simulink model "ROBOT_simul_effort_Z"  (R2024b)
settings: Solver=VariableStepAuto  StartTime=0.0  StopTime=5  RelTol=1e-3
undefined symbols (not defined in the file): a, ARRIERE_Defaut_sldprt, avant01_Defaut_sldprt, avant02_Defaut_sldprt, avant03_Defaut_sldprt, avant1_Defaut_sldprt, AXE, BASE_Defaut_sldprt, BIELLE, BIELLE_Defaut_sldprt, BRAS_Defaut_sldprt, bras_Defaut_sldprt, C_Realiste_sldprt, CABLE_Defaut_sldprt, cable_Defaut_sldprt, CACHE_Defaut_sldprt, CARTE, carte_Defaut_sldprt, CARTER, carter, CHC, CODEUR_Defaut_sldprt, cruciforme, cylindrique, deg, Drive, Fichiers, Fichiers_Matlab_sujetA, FIXATION, fixation_Defaut_sldprt, H, HEXAGONALE_Defaut_sldprt, joint_Defaut_sldprt, kg, m, M4, M4_Defaut_sldprt, manette1_Defaut_sldprt, manette2_Defaut_sldprt, MATLAB, Matlab, matlab_Defaut_sldprt, mm, modif, MOTEUR_Defaut_sldprt, N, NEZ_Defaut_sldprt, nom, palier, PARALLELOGRAMME_Defaut_sldprt, petite, plaque, rad, Ressort, Rondelle, ROTOR_Defaut_sldprt, s, SET, simple, socle_Defaut_sldprt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
libraries: sm_lib x463, fl_lib x45, nesl_utility x27, simulink x2
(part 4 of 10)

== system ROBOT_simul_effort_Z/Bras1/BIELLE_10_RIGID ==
  AXE_BIELLE_1_RIGID : Subsystem
  AXE_BIELLE_2_RIGID : Subsystem
  BIELLE_PARALLELOGRAMME_1_RIGID : Subsystem
  ReferenceFrame : sm_lib/Frames and Transforms/Reference Frame
  Transform : sm_lib/Frames and Transforms/Rigid Transform  RotationMethod=ArbitraryAxis  FollAlignAxisA=+X  BaseAlignAxisA=+Y  FollAlignAxisB=+Y  BaseAlignAxisB=+Z  RotationStandardAxis=+Z  RotationAngle=2.0943951023931957  RotationAngleUnits=rad  RotationArbitraryAxis=[0.57735026918962573 -0.57735026918962573 0.57735026918962562]  RotationSequenceAxes=FollowerAxes  RotationSequence=XYX  RotationSequenceAngles=[0 0 0]  RotationSequenceAnglesUnits=deg  RotationMatrix=[1 0 0; 0 1 0; 0 0 1]  Quaternion=[1 0 0 0]  TranslationMethod=Cartesian  TranslationCartesianOffset=[-181.1287710013672 12.999999999999993 -105.75000000000001]  TranslationCartesianOffsetUnits=mm  TranslationStandardAxis=+Z  TranslationStandardOffset=0  TranslationStandardOffsetUnits=mm  TranslationROffset=0  TranslationROffsetUnits=m  TranslationThetaOffset=0  TranslationThetaOffsetUnits=deg  TranslationZOffset=0  TranslationZOffsetUnits=m
  Transform1 : sm_lib/Frames and Transforms/Rigid Transform  RotationMethod=ArbitraryAxis  FollAlignAxisA=+X  BaseAlignAxisA=+Y  FollAlignAxisB=+Y  BaseAlignAxisB=+Z  RotationStandardAxis=+Z  RotationAngle=2.0943951023931953  RotationAngleUnits=rad  RotationArbitraryAxis=[0.57735026918962584 -0.57735026918962584 0.57735026918962584]  RotationSequenceAxes=FollowerAxes  RotationSequence=XYX  RotationSequenceAngles=[0 0 0]  RotationSequenceAnglesUnits=deg  RotationMatrix=[1 0 0; 0 1 0; 0 0 1]  Quaternion=[1 0 0 0]  TranslationMethod=Cartesian  TranslationCartesianOffset=[-181.12877100136717 13.000000000000004 -3.249999999999996]  TranslationCartesianOffsetUnits=mm  TranslationStandardAxis=+Z  TranslationStandardOffset=0  TranslationStandardOffsetUnits=mm  TranslationROffset=0  TranslationROffsetUnits=m  TranslationThetaOffset=0  TranslationThetaOffsetUnits=deg  TranslationZOffset=0  TranslationZOffsetUnits=m
  Transform2 : sm_lib/Frames and Transforms/Rigid Transform  RotationMethod=ArbitraryAxis  FollAlignAxisA=+X  BaseAlignAxisA=+Y  FollAlignAxisB=+Y  BaseAlignAxisB=+Z  RotationStandardAxis=+Z  RotationAngle=3.1415926535897931  RotationAngleUnits=rad  RotationArbitraryAxis=[-0.70710678118654746 0.70710678118654768 0]  RotationSequenceAxes=FollowerAxes  RotationSequence=XYX  RotationSequenceAngles=[0 0 0]  RotationSequenceAnglesUnits=deg  RotationMatrix=[1 0 0; 0 1 0; 0 0 1]  Quaternion=[1 0 0 0]  TranslationMethod=Cartesian  TranslationCartesianOffset=[-178.12877100136717 5.0000000000000115 -54.500000000000007]  TranslationCartesianOffsetUnits=mm  TranslationStandardAxis=+Z  TranslationStandardOffset=0  TranslationStandardOffsetUnits=mm  TranslationROffset=0  TranslationROffsetUnits=m  TranslationThetaOffset=0  TranslationThetaOffsetUnits=deg  TranslationZOffset=0  TranslationZOffsetUnits=m
  Transform3 : sm_lib/Frames and Transforms/Rigid Transform  RotationMethod=ArbitraryAxis  FollAlignAxisA=+X  BaseAlignAxisA=+Y  FollAlignAxisB=+Y  BaseAlignAxisB=+Z  RotationStandardAxis=+Z  RotationAngle=1.7602050674842988  RotationAngleUnits=rad  RotationArbitraryAxis=[-0.82650316451596495 -0.3980530863120495 -0.3980530863120495]  RotationSequenceAxes=FollowerAxes  RotationSequence=XYX  RotationSequenceAngles=[0 0 0]  RotationSequenceAnglesUnits=deg  RotationMatrix=[1 0 0; 0 1 0; 0 0 1]  Quaternion=[1 0 0 0]  TranslationMethod=Cartesian  TranslationCartesianOffset=[-181.1287710013672 4.999999999999984 -105.75000000000001]  TranslationCartesianOffsetUnits=mm  TranslationStandardAxis=+Z  TranslationStandardOffset=0  TranslationStandardOffsetUnits=mm  TranslationROffset=0  TranslationROffsetUnits=m  TranslationThetaOffset=0  TranslationThetaOffsetUnits=deg  TranslationZOffset=0  TranslationZOffsetUnits=m
  Transform4 : sm_lib/Frames and Transforms/Rigid Transform  RotationMethod=ArbitraryAxis  FollAlignAxisA=+X  BaseAlignAxisA=+Y  FollAlignAxisB=+Y  BaseAlignAxisB=+Z  RotationStandardAxis=+Z  RotationAngle=1.7602050674842997  RotationAngleUnits=rad  RotationArbitraryAxis=[-0.82650316451596506 -0.39805308631204933 -0.39805308631204933]  RotationSequenceAxes=FollowerAxes  RotationSequence=XYX  RotationSequenceAngles=[0 0 0]  RotationSequenceAnglesUnits=deg  RotationMatrix=[1 0 0; 0 1 0; 0 0 1]  Quaternion=[1 0 0 0]  TranslationMethod=Cartesian  TranslationCartesianOffset=[-181.12877100136717 5.0000000000000115 -3.249999999999996]  TranslationCartesianOffsetUnits=mm  TranslationStandardAxis=+Z  TranslationStandardOffset=0  TranslationStandardOffsetUnits=mm  TranslationROffset=0  TranslationROffsetUnits=m  TranslationThetaOffset=0  TranslationThetaOffsetUnits=deg  TranslationZOffset=0  TranslationZOffsetUnits=m
  F1 : PMIOPort  Side=Right
  F : PMIOPort  Port=2  Side=Left
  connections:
  Transform/LConn1 -- ReferenceFrame/RConn1 -- Transform3/LConn1 -- Transform4/LConn1 -- Transform2/LConn1 -- Transform1/LConn1
  Transform/RConn1 -- F/RConn1
  Transform1/RConn1 -- F1/RConn1
  BIELLE_PARALLELOGRAMME_1_RIGID/LConn1 -- Transform2/RConn1
  AXE_BIELLE_1_RIGID/LConn1 -- Transform3/RConn1
  AXE_BIELLE_2_RIGID/LConn1 -- Transform4/RConn1

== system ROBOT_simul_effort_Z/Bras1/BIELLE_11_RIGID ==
  AXE_BIELLE_1_RIGID : Subsystem
  AXE_BIELLE_2_RIGID : Subsystem
  BIELLE_PARALLELOGRAMME_1_RIGID : Subsystem
  ReferenceFrame : sm_lib/Frames and Transforms/Reference Frame
  Transform : sm_lib/Frames and Transforms/Rigid Transform  RotationMethod=ArbitraryAxis  FollAlignAxisA=+X  BaseAlignAxisA=+Y  FollAlignAxisB=+Y  BaseAlignAxisB=+Z  RotationStandardAxis=+Z  RotationAngle=2.0943951023931962  RotationAngleUnits=rad  RotationArbitraryAxis=[0.57735026918962595 -0.57735026918962562 0.57735026918962562]  RotationSequenceAxes=FollowerAxes  RotationSequence=XYX  RotationSequenceAngles=[0 0 0]  RotationSequenceAnglesUnits=deg  RotationMatrix=[1 0 0; 0 1 0; 0 0 1]  Quaternion=[1 0 0 0]  TranslationMethod=Cartesian  TranslationCartesianOffset=[-181.12877100136717 13.000000000000018 -105.75000000000001]  TranslationCartesianOffsetUnits=mm  TranslationStandardAxis=+Z  TranslationStandardOffset=0  TranslationStandardOffsetUnits=mm  TranslationROffset=0  TranslationROffsetUnits=m  TranslationThetaOffset=0  TranslationThetaOffsetUnits=deg  TranslationZOffset=0  TranslationZOffsetUnits=m
  Transform1 : sm_lib/Frames and Transforms/Rigid Transform  RotationMethod=ArbitraryAxis  FollAlignAxisA=+X  BaseAlignAxisA=+Y  FollAlignAxisB=+Y  BaseAlignAxisB=+Z  RotationStandardAxis=+Z  RotationAngle=2.0943951023931957  RotationAngleUnits=rad  RotationArbitraryAxis=[0.57735026918962573 -0.57735026918962562 0.57735026918962595]  RotationSequenceAxes=FollowerAxes  RotationSequence=XYX  RotationSequenceAngles=[0 0 0]  RotationSequenceAnglesUnits=deg  RotationMatrix=[1 0 0; 0 1 0; 0 0 1]  Quaternion=[1 0 0 0]  TranslationMethod=Cartesian  TranslationCartesianOffset=[-181.12877100136714 13.000000000000014 -3.2499999999999889]  TranslationCartesianOffsetUnits=mm  TranslationStandardAxis=+Z  TranslationStandardOffset=0  TranslationStandardOffsetUnits=mm  TranslationROffset=0  TranslationROffsetUnits=m  TranslationThetaOffset=0  TranslationThetaOffsetUnits=deg  TranslationZOffset=0  TranslationZOffsetUnits=m
  Transform2 : sm_lib/Frames and Transforms/Rigid Transform  RotationMethod=ArbitraryAxis  FollAlignAxisA=+X  BaseAlignAxisA=+Y  FollAlignAxisB=+Y  BaseAlignAxisB=+Z  RotationStandardAxis=+Z  RotationAngle=3.1415926535897931  RotationAngleUnits=rad  RotationArbitraryAxis=[-0.70710678118654746 0.70710678118654757 0]  RotationSequenceAxes=FollowerAxes  RotationSequence=XYX  RotationSequenceAngles=[0 0 0]  RotationSequenceAnglesUnits=deg  RotationMatrix=[1 0 0; 0 1 0; 0 0 1]  Quaternion=[1 0 0 0]  TranslationMethod=Cartesian  TranslationCartesianOffset=[-178.12877100136714 5.0000000000000044 -54.500000000000007]  TranslationCartesianOffsetUnits=mm  TranslationStandardAxis=+Z  TranslationStandardOffset=0  TranslationStandardOffsetUnits=mm  TranslationROffset=0  TranslationROffsetUnits=m  TranslationThetaOffset=0  TranslationThetaOffsetUnits=deg  TranslationZOffset=0  TranslationZOffsetUnits=m
  Transform3 : sm_lib/Frames and Transforms/Rigid Transform  RotationMethod=ArbitraryAxis  FollAlignAxisA=+X  BaseAlignAxisA=+Y  FollAlignAxisB=+Y  BaseAlignAxisB=+Z  RotationStandardAxis=+Z  RotationAngle=1.7602050674842991  RotationAngleUnits=rad  RotationArbitraryAxis=[-0.82650316451596495 -0.3980530863120495 -0.39805308631204944]  RotationSequenceAxes=FollowerAxes  RotationSequence=XYX  RotationSequenceAngles=[0 0 0]  RotationSequenceAnglesUnits=deg  RotationMatrix=[1 0 0; 0 1 0; 0 0 1]  Quaternion=[1 0 0 0]  TranslationMethod=Cartesian  TranslationCartesianOffset=[-181.12877100136717 5.0000000000000044 -105.75000000000001]  TranslationCartesianOffsetUnits=mm  TranslationStandardAxis=+Z  TranslationStandardOffset=0  TranslationStandardOffsetUnits=mm  TranslationROffset=0  TranslationROffsetUnits=m  TranslationThetaOffset=0  TranslationThetaOffsetUnits=deg  TranslationZOffset=0  TranslationZOffsetUnits=m
  Transform4 : sm_lib/Frames and Transforms/Rigid Transform  RotationMethod=ArbitraryAxis  FollAlignAxisA=+X  BaseAlignAxisA=+Y  FollAlignAxisB=+Y  BaseAlignAxisB=+Z  RotationStandardAxis=+Z  RotationAngle=1.7602050674842995  RotationAngleUnits=rad  RotationArbitraryAxis=[-0.82650316451596506 -0.39805308631204939 -0.39805308631204933]  RotationSequenceAxes=FollowerAxes  RotationSequence=XYX  RotationSequenceAngles=[0 0 0]  RotationSequenceAnglesUnits=deg  RotationMatrix=[1 0 0; 0 1 0; 0 0 1]  Quaternion=[1 0 0 0]  TranslationMethod=Cartesian  TranslationCartesianOffset=[-181.12877100136714 5.0000000000000044 -3.2499999999999889]  TranslationCartesianOffsetUnits=mm  TranslationStandardAxis=+Z  TranslationStandardOffset=0  TranslationStandardOffsetUnits=mm  TranslationROffset=0  TranslationROffsetUnits=m  TranslationThetaOffset=0  TranslationThetaOffsetUnits=deg  TranslationZOffset=0  TranslationZOffsetUnits=m
  F1 : PMIOPort  Side=Right
  F : PMIOPort  Port=2  Side=Left
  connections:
  Transform/LConn1 -- ReferenceFrame/RConn1 -- Transform3/LConn1 -- Transform4/LConn1 -- Transform2/LConn1 -- Transform1/LConn1
  Transform/RConn1 -- F/RConn1
  Transform1/RConn1 -- F1/RConn1
  BIELLE_PARALLELOGRAMME_1_RIGID/LConn1 -- Transform2/RConn1
  AXE_BIELLE_1_RIGID/LConn1 -- Transform3/RConn1
  AXE_BIELLE_2_RIGID/LConn1 -- Transform4/RConn1

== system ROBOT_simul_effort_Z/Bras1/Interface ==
  Angular Velocity Source : fl_lib/Mechanical/Mechanical Sources/Ideal Angular Velocity Source
  Torque Sensor : fl_lib/Mechanical/Mechanical Sensors/Ideal Torque Sensor
  C : PMIOPort  Side=Left
  T : PMIOPort  Port=2  Side=Right
  w : PMIOPort  Port=3  Side=Right
  R : PMIOPort  Port=4  Side=Left
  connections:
  R/RConn1 -- Angular Velocity Source/LConn1
  Torque Sensor/LConn1 -- Angular Velocity Source/RConn2
  Torque Sensor/RConn2 -- T/RConn1
  C/RConn1 -- Torque Sensor/RConn1
  Angular Velocity Source/RConn1 -- w/RConn1

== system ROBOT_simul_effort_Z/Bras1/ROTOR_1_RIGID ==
  CODEUR_1_RIGID : Subsystem
  ROTOR_1_RIGID : Subsystem
  ReferenceFrame : sm_lib/Frames and Transforms/Reference Frame
  Transform : sm_lib/Frames and Transforms/Rigid Transform  RotationMethod=ArbitraryAxis  FollAlignAxisA=+X  BaseAlignAxisA=+Y  FollAlignAxisB=+Y  BaseAlignAxisB=+Z  RotationStandardAxis=+Z  RotationAngle=2.0943951023931953  RotationAngleUnits=rad  RotationArbitraryAxis=[0.57735026918962595 0.57735026918962562 0.57735026918962562]  RotationSequenceAxes=FollowerAxes  RotationSequence=XYX  RotationSequenceAngles=[0 0 0]  RotationSequenceAnglesUnits=deg  RotationMatrix=[1 0 0; 0 1 0; 0 0 1]  Quaternion=[1 0 0 0]  TranslationMethod=Cartesian  TranslationCartesianOffset=[29.900000000000013 -3.5527136788005009e-15 2.2204460492503131e-14]  TranslationCartesianOffsetUnits=mm  TranslationStandardAxis=+Z  TranslationStandardOffset=0  TranslationStandardOffsetUnits=mm  TranslationROffset=0  TranslationROffsetUnits=m  TranslationThetaOffset=0  TranslationThetaOffsetUnits=deg  TranslationZOffset=0  TranslationZOffsetUnits=m
  Transform1 : sm_lib/Frames and Transforms/Rigid Transform  RotationMethod=ArbitraryAxis  FollAlignAxisA=+X  BaseAlignAxisA=+Y  FollAlignAxisB=+Y  BaseAlignAxisB=+Z  RotationStandardAxis=+Z  RotationAngle=1.9381695666920586  RotationAngleUnits=rad  RotationArbitraryAxis=[0.51405666735189148 -0.51405666735189148 0.68665237602598705]  RotationSequenceAxes=FollowerAxes  RotationSequence=XYX  RotationSequenceAngles=[0 0 0]  RotationSequenceAnglesUnits=deg  RotationMatrix=[1 0 0; 0 1 0; 0 0 1]  Quaternion=[1 0 0 0]  TranslationMethod=Cartesian  TranslationCartesianOffset=[30.899999999999981 0 0]  TranslationCartesianOffsetUnits=mm  TranslationStandardAxis=+Z  TranslationStandardOffset=0  TranslationStandardOffsetUnits=mm  TranslationROffset=0  TranslationROffsetUnits=m  TranslationThetaOffset=0  TranslationThetaOffsetUnits=deg  TranslationZOffset=0  TranslationZOffsetUnits=m
  Transform2 : sm_lib/Frames and Transforms/Rigid Transform  RotationMethod=ArbitraryAxis  FollAlignAxisA=+X  BaseAlignAxisA=+Y  FollAlignAxisB=+Y  BaseAlignAxisB=+Z  RotationStandardAxis=+Z  RotationAngle=1.624664356272121  RotationAngleUnits=rad  RotationArbitraryAxis=[-0.22603347840136145 0.22603347840136123 0.94753244444903439]  RotationSequenceAxes=FollowerAxes  RotationSequence=XYX  RotationSequenceAngles=[0 0 0]  RotationSequenceAnglesUnits=deg  RotationMatrix=[1 0 0; 0 1 0; 0 0 1]  Quaternion=[1 0 0 0]  TranslationMethod=Cartesian  TranslationCartesianOffset=[-36.399999999999999 0 0]  TranslationCartesianOffsetUnits=mm  TranslationStandardAxis=+Z  TranslationStandardOffset=0  TranslationStandardOffsetUnits=mm  TranslationROffset=0  TranslationROffsetUnits=m  TranslationThetaOffset=0  TranslationThetaOffsetUnits=deg  TranslationZOffset=0  TranslationZOffsetUnits=m
  F : PMIOPort  Side=Left
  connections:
  Transform/LConn1 -- ReferenceFrame/RConn1 -- Transform1/LConn1 -- Transform2/LConn1
  Transform/RConn1 -- F/RConn1
  ROTOR_1_RIGID/LConn1 -- Transform1/RConn1
  CODEUR_1_RIGID/LConn1 -- Transform2/RConn1

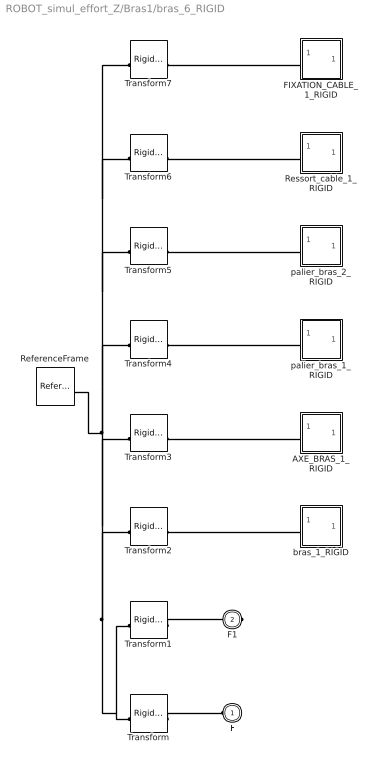
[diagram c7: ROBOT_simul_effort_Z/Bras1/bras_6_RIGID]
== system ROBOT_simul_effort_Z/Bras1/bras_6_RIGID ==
  AXE_BRAS_1_RIGID : Subsystem
  FIXATION_CABLE_1_RIGID : Subsystem
  ReferenceFrame : sm_lib/Frames and Transforms/Reference Frame
  Ressort_cable_1_RIGID : Subsystem
  Transform : sm_lib/Frames and Transforms/Rigid Transform  RotationMethod=ArbitraryAxis  FollAlignAxisA=+X  BaseAlignAxisA=+Y  FollAlignAxisB=+Y  BaseAlignAxisB=+Z  RotationStandardAxis=+Z  RotationAngle=2.0943951023931957  RotationAngleUnits=rad  RotationArbitraryAxis=[-0.57735026918962551 -0.57735026918962595 0.57735026918962573]  RotationSequenceAxes=FollowerAxes  RotationSequence=XYX  RotationSequenceAngles=[0 0 0]  RotationSequenceAnglesUnits=deg  RotationMatrix=[1 0 0; 0 1 0; 0 0 1]  Quaternion=[1 0 0 0]  TranslationMethod=Cartesian  TranslationCartesianOffset=[-97.415569487383038 39.82561820207529 -20.980989744699272]  TranslationCartesianOffsetUnits=mm  TranslationStandardAxis=+Z  TranslationStandardOffset=0  TranslationStandardOffsetUnits=mm  TranslationROffset=0  TranslationROffsetUnits=m  TranslationThetaOffset=0  TranslationThetaOffsetUnits=deg  TranslationZOffset=0  TranslationZOffsetUnits=m
  Transform1 : sm_lib/Frames and Transforms/Rigid Transform  RotationMethod=ArbitraryAxis  FollAlignAxisA=+X  BaseAlignAxisA=+Y  FollAlignAxisB=+Y  BaseAlignAxisB=+Z  RotationStandardAxis=+Z  RotationAngle=2.0943951023931953  RotationAngleUnits=rad  RotationArbitraryAxis=[0.57735026918962584 0.57735026918962584 0.57735026918962584]  RotationSequenceAxes=FollowerAxes  RotationSequence=XYX  RotationSequenceAngles=[0 0 0]  RotationSequenceAnglesUnits=deg  RotationMatrix=[1 0 0; 0 1 0; 0 0 1]  Quaternion=[1 0 0 0]  TranslationMethod=Cartesian  TranslationCartesianOffset=[-176.59192436800635 99.825618202078147 -20.980989744703663]  TranslationCartesianOffsetUnits=mm  TranslationStandardAxis=+Z  TranslationStandardOffset=0  TranslationStandardOffsetUnits=mm  TranslationROffset=0  TranslationROffsetUnits=m  TranslationThetaOffset=0  TranslationThetaOffsetUnits=deg  TranslationZOffset=0  TranslationZOffsetUnits=m
  Transform2 : sm_lib/Frames and Transforms/Rigid Transform  RotationMethod=ArbitraryAxis  FollAlignAxisA=+X  BaseAlignAxisA=+Y  FollAlignAxisB=+Y  BaseAlignAxisB=+Z  RotationStandardAxis=+Z  RotationAngle=1.5707963267948968  RotationAngleUnits=rad  RotationArbitraryAxis=[-0 -1 -0]  RotationSequenceAxes=FollowerAxes  RotationSequence=XYX  RotationSequenceAngles=[0 0 0]  RotationSequenceAnglesUnits=deg  RotationMatrix=[1 0 0; 0 1 0; 0 0 1]  Quaternion=[1 0 0 0]  TranslationMethod=Cartesian  TranslationCartesianOffset=[-166.59192436800635 39.825618202078147 -20.98098974470366]  TranslationCartesianOffsetUnits=mm  TranslationStandardAxis=+Z  TranslationStandardOffset=0  TranslationStandardOffsetUnits=mm  TranslationROffset=0  TranslationROffsetUnits=m  TranslationThetaOffset=0  TranslationThetaOffsetUnits=deg  TranslationZOffset=0  TranslationZOffsetUnits=m
  Transform3 : sm_lib/Frames and Transforms/Rigid Transform  RotationMethod=ArbitraryAxis  FollAlignAxisA=+X  BaseAlignAxisA=+Y  FollAlignAxisB=+Y  BaseAlignAxisB=+Z  RotationStandardAxis=+Z  RotationAngle=1.5707963267948968  RotationAngleUnits=rad  RotationArbitraryAxis=[0 1 0]  RotationSequenceAxes=FollowerAxes  RotationSequence=XYX  RotationSequenceAngles=[0 0 0]  RotationSequenceAnglesUnits=deg  RotationMatrix=[1 0 0; 0 1 0; 0 0 1]  Quaternion=[1 0 0 0]  TranslationMethod=Cartesian  TranslationCartesianOffset=[-166.59192436800635 39.825618202078147 -20.98098974470366]  TranslationCartesianOffsetUnits=mm  TranslationStandardAxis=+Z  TranslationStandardOffset=0  TranslationStandardOffsetUnits=mm  TranslationROffset=0  TranslationROffsetUnits=m  TranslationThetaOffset=0  TranslationThetaOffsetUnits=deg  TranslationZOffset=0  TranslationZOffsetUnits=m
  Transform4 : sm_lib/Frames and Transforms/Rigid Transform  RotationMethod=None  FollAlignAxisA=+X  BaseAlignAxisA=+Y  FollAlignAxisB=+Y  BaseAlignAxisB=+Z  RotationStandardAxis=+Z  RotationAngle=0  RotationAngleUnits=deg  RotationArbitraryAxis=[0 0 1]  RotationSequenceAxes=FollowerAxes  RotationSequence=XYX  RotationSequenceAngles=[0 0 0]  RotationSequenceAnglesUnits=deg  RotationMatrix=[1 0 0; 0 1 0; 0 0 1]  Quaternion=[1 0 0 0]  TranslationMethod=None  TranslationCartesianOffset=[0 0 0]  TranslationCartesianOffsetUnits=m  TranslationStandardAxis=+Z  TranslationStandardOffset=0  TranslationStandardOffsetUnits=m  TranslationROffset=0  TranslationROffsetUnits=m  TranslationThetaOffset=0  TranslationThetaOffsetUnits=deg  TranslationZOffset=0  TranslationZOffsetUnits=m
  Transform5 : sm_lib/Frames and Transforms/Rigid Transform  RotationMethod=ArbitraryAxis  FollAlignAxisA=+X  BaseAlignAxisA=+Y  FollAlignAxisB=+Y  BaseAlignAxisB=+Z  RotationStandardAxis=+Z  RotationAngle=3.1415926535897931  RotationAngleUnits=rad  RotationArbitraryAxis=[0 0.83121877946981937 -0.55594544755461728]  RotationSequenceAxes=FollowerAxes  RotationSequence=XYX  RotationSequenceAngles=[0 0 0]  RotationSequenceAnglesUnits=deg  RotationMatrix=[1 0 0; 0 1 0; 0 0 1]  Quaternion=[1 0 0 0]  TranslationMethod=Cartesian  TranslationCartesianOffset=[-333.18384873601275 5.2270863233389582 7.8152493791980238]  TranslationCartesianOffsetUnits=mm  TranslationStandardAxis=+Z  TranslationStandardOffset=0  TranslationStandardOffsetUnits=mm  TranslationROffset=0  TranslationROffsetUnits=m  TranslationThetaOffset=0  TranslationThetaOffsetUnits=deg  TranslationZOffset=0  TranslationZOffsetUnits=m
  Transform6 : sm_lib/Frames and Transforms/Rigid Transform  RotationMethod=ArbitraryAxis  FollAlignAxisA=+X  BaseAlignAxisA=+Y  FollAlignAxisB=+Y  BaseAlignAxisB=+Z  RotationStandardAxis=+Z  RotationAngle=1.5707963267948968  RotationAngleUnits=rad  RotationArbitraryAxis=[1 0 0]  RotationSequenceAxes=FollowerAxes  RotationSequence=XYX  RotationSequenceAngles=[0 0 0]  RotationSequenceAnglesUnits=deg  RotationMatrix=[1 0 0; 0 1 0; 0 0 1]  Quaternion=[1 0 0 0]  TranslationMethod=Cartesian  TranslationCartesianOffset=[-166.59192436800637 17.182941135267072 -24.980989744703663]  TranslationCartesianOffsetUnits=mm  TranslationStandardAxis=+Z  TranslationStandardOffset=0  TranslationStandardOffsetUnits=mm  TranslationROffset=0  TranslationROffsetUnits=m  TranslationThetaOffset=0  TranslationThetaOffsetUnits=deg  TranslationZOffset=0  TranslationZOffsetUnits=m
  Transform7 : sm_lib/Frames and Transforms/Rigid Transform  RotationMethod=ArbitraryAxis  FollAlignAxisA=+X  BaseAlignAxisA=+Y  FollAlignAxisB=+Y  BaseAlignAxisB=+Z  RotationStandardAxis=+Z  RotationAngle=1.0159852938148253  RotationAngleUnits=rad  RotationArbitraryAxis=[-1 0 0]  RotationSequenceAxes=FollowerAxes  RotationSequence=XYX  RotationSequenceAngles=[0 0 0]  RotationSequenceAnglesUnits=deg  RotationMatrix=[1 0 0; 0 1 0; 0 0 1]  Quaternion=[1 0 0 0]  TranslationMethod=Cartesian  TranslationCartesianOffset=[-172.59192436800637 90.586314327933906 3.4188407632840327]  TranslationCartesianOffsetUnits=mm  TranslationStandardAxis=+Z  TranslationStandardOffset=0  TranslationStandardOffsetUnits=mm  TranslationROffset=0  TranslationROffsetUnits=m  TranslationThetaOffset=0  TranslationThetaOffsetUnits=deg  TranslationZOffset=0  TranslationZOffsetUnits=m
  bras_1_RIGID : Subsystem
  palier_bras_1_RIGID : Subsystem
  palier_bras_2_RIGID : Subsystem
  F : PMIOPort  Side=Left
  F1 : PMIOPort  Port=2  Side=Right
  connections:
  Transform/LConn1 -- ReferenceFrame/RConn1 -- Transform6/LConn1 -- Transform7/LConn1 -- Transform5/LConn1 -- Transform4/LConn1 -- Transform3/LConn1 -- Transform2/LConn1 -- Transform1/LConn1
  Transform/RConn1 -- F/RConn1
  Transform1/RConn1 -- F1/RConn1
  Transform2/RConn1 -- bras_1_RIGID/LConn1
  AXE_BRAS_1_RIGID/LConn1 -- Transform3/RConn1
  Transform4/RConn1 -- palier_bras_1_RIGID/LConn1
  Transform5/RConn1 -- palier_bras_2_RIGID/LConn1
  Ressort_cable_1_RIGID/LConn1 -- Transform6/RConn1
  FIXATION_CABLE_1_RIGID/LConn1 -- Transform7/RConn1

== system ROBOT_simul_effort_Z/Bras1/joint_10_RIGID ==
  AXE_BRAS_1_RIGID : Subsystem
  ReferenceFrame : sm_lib/Frames and Transforms/Reference Frame
  Transform : sm_lib/Frames and Transforms/Rigid Transform  RotationMethod=ArbitraryAxis  FollAlignAxisA=+X  BaseAlignAxisA=+Y  FollAlignAxisB=+Y  BaseAlignAxisB=+Z  RotationStandardAxis=+Z  RotationAngle=1.9754511492118261  RotationAngleUnits=rad  RotationArbitraryAxis=[-0.53149434051907762 -0.53149434051907807 -0.65956616953295977]  RotationSequenceAxes=FollowerAxes  RotationSequence=XYX  RotationSequenceAngles=[0 0 0]  RotationSequenceAnglesUnits=deg  RotationMatrix=[1 0 0; 0 1 0; 0 0 1]  Quaternion=[1 0 0 0]  TranslationMethod=Cartesian  TranslationCartesianOffset=[-153.62772197331242 116.19029839316632 -133.8263224253264]  TranslationCartesianOffsetUnits=mm  TranslationStandardAxis=+Z  TranslationStandardOffset=0  TranslationStandardOffsetUnits=mm  TranslationROffset=0  TranslationROffsetUnits=m  TranslationThetaOffset=0  TranslationThetaOffsetUnits=deg  TranslationZOffset=0  TranslationZOffsetUnits=m
  Transform1 : sm_lib/Frames and Transforms/Rigid Transform  RotationMethod=ArbitraryAxis  FollAlignAxisA=+X  BaseAlignAxisA=+Y  FollAlignAxisB=+Y  BaseAlignAxisB=+Z  RotationStandardAxis=+Z  RotationAngle=2.2221940470110657  RotationAngleUnits=rad  RotationArbitraryAxis=[0.61437017396793003 -0.61437017396792981 0.49507431631749077]  RotationSequenceAxes=FollowerAxes  RotationSequence=XYX  RotationSequenceAngles=[0 0 0]  RotationSequenceAnglesUnits=deg  RotationMatrix=[1 0 0; 0 1 0; 0 0 1]  Quaternion=[1 0 0 0]  TranslationMethod=Cartesian  TranslationCartesianOffset=[-181.62772197331248 131.82453775326121 -130.42476989284125]  TranslationCartesianOffsetUnits=mm  TranslationStandardAxis=+Z  TranslationStandardOffset=0  TranslationStandardOffsetUnits=mm  TranslationROffset=0  TranslationROffsetUnits=m  TranslationThetaOffset=0  TranslationThetaOffsetUnits=deg  TranslationZOffset=0  TranslationZOffsetUnits=m
  Transform2 : sm_lib/Frames and Transforms/Rigid Transform  RotationMethod=ArbitraryAxis  FollAlignAxisA=+X  BaseAlignAxisA=+Y  FollAlignAxisB=+Y  BaseAlignAxisB=+Z  RotationStandardAxis=+Z  RotationAngle=2.0943951023931957  RotationAngleUnits=rad  RotationArbitraryAxis=[0.57735026918962551 0.57735026918962584 0.57735026918962595]  RotationSequenceAxes=FollowerAxes  RotationSequence=XYX  RotationSequenceAngles=[0 0 0]  RotationSequenceAnglesUnits=deg  RotationMatrix=[1 0 0; 0 1 0; 0 0 1]  Quaternion=[1 0 0 0]  TranslationMethod=Cartesian  TranslationCartesianOffset=[-177.62772197331233 126.39913469761095 -143.1183707091472]  TranslationCartesianOffsetUnits=mm  TranslationStandardAxis=+Z  TranslationStandardOffset=0  TranslationStandardOffsetUnits=mm  TranslationROffset=0  TranslationROffsetUnits=m  TranslationThetaOffset=0  TranslationThetaOffsetUnits=deg  TranslationZOffset=0  TranslationZOffsetUnits=m
  Transform3 : sm_lib/Frames and Transforms/Rigid Transform  RotationMethod=ArbitraryAxis  FollAlignAxisA=+X  BaseAlignAxisA=+Y  FollAlignAxisB=+Y  BaseAlignAxisB=+Z  RotationStandardAxis=+Z  RotationAngle=1.7850283121554718  RotationAngleUnits=rad  RotationArbitraryAxis=[1 7.8579866763579256e-16 -6.7960803884612889e-16]  RotationSequenceAxes=FollowerAxes  RotationSequence=XYX  RotationSequenceAngles=[0 0 0]  RotationSequenceAnglesUnits=deg  RotationMatrix=[1 0 0; 0 1 0; 0 0 1]  Quaternion=[1 0 0 0]  TranslationMethod=Cartesian  TranslationCartesianOffset=[-167.62772197331245 128.09991096385986 -150.93549038919826]  TranslationCartesianOffsetUnits=mm  TranslationStandardAxis=+Z  TranslationStandardOffset=0  TranslationStandardOffsetUnits=mm  TranslationROffset=0  TranslationROffsetUnits=m  TranslationThetaOffset=0  TranslationThetaOffsetUnits=deg  TranslationZOffset=0  TranslationZOffsetUnits=m
  Transform4 : sm_lib/Frames and Transforms/Rigid Transform  RotationMethod=ArbitraryAxis  FollAlignAxisA=+X  BaseAlignAxisA=+Y  FollAlignAxisB=+Y  BaseAlignAxisB=+Z  RotationStandardAxis=+Z  RotationAngle=1.5707963267948968  RotationAngleUnits=rad  RotationArbitraryAxis=[-0 -1 -0]  RotationSequenceAxes=FollowerAxes  RotationSequence=XYX  RotationSequenceAngles=[0 0 0]  RotationSequenceAnglesUnits=deg  RotationMatrix=[1 0 0; 0 1 0; 0 0 1]  Quaternion=[1 0 0 0]  TranslationMethod=Cartesian  TranslationCartesianOffset=[-167.62772197331239 126.39913469761737 -143.11837070915072]  TranslationCartesianOffsetUnits=mm  TranslationStandardAxis=+Z  TranslationStandardOffset=0  TranslationStandardOffsetUnits=mm  TranslationROffset=0  TranslationROffsetUnits=m  TranslationThetaOffset=0  TranslationThetaOffsetUnits=deg  TranslationZOffset=0  TranslationZOffsetUnits=m
  joint_1_RIGID : Subsystem
  F2 : PMIOPort  Side=Left
  F1 : PMIOPort  Port=2  Side=Right
  F : PMIOPort  Port=3  Side=Right
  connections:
  Transform/LConn1 -- ReferenceFrame/RConn1 -- Transform3/LConn1 -- Transform4/LConn1 -- Transform2/LConn1 -- Transform1/LConn1
  Transform/RConn1 -- F/RConn1
  Transform1/RConn1 -- F1/RConn1
  Transform2/RConn1 -- F2/RConn1
  Transform3/RConn1 -- joint_1_RIGID/LConn1
  AXE_BRAS_1_RIGID/LConn1 -- Transform4/RConn1

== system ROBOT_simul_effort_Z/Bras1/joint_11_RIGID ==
  AXE_BRAS_1_RIGID : Subsystem
  ReferenceFrame : sm_lib/Frames and Transforms/Reference Frame
  Transform : sm_lib/Frames and Transforms/Rigid Transform  RotationMethod=ArbitraryAxis  FollAlignAxisA=+X  BaseAlignAxisA=+Y  FollAlignAxisB=+Y  BaseAlignAxisB=+Z  RotationStandardAxis=+Z  RotationAngle=2.2221940470110675  RotationAngleUnits=rad  RotationArbitraryAxis=[0.61437017396793037 -0.61437017396793037 0.49507431631748977]  RotationSequenceAxes=FollowerAxes  RotationSequence=XYX  RotationSequenceAngles=[0 0 0]  RotationSequenceAnglesUnits=deg  RotationMatrix=[1 0 0; 0 1 0; 0 0 1]  Quaternion=[1 0 0 0]  TranslationMethod=Cartesian  TranslationCartesianOffset=[-153.62772197331219 131.82453775326144 -130.42476989284148]  TranslationCartesianOffsetUnits=mm  TranslationStandardAxis=+Z  TranslationStandardOffset=0  TranslationStandardOffsetUnits=mm  TranslationROffset=0  TranslationROffsetUnits=m  TranslationThetaOffset=0  TranslationThetaOffsetUnits=deg  TranslationZOffset=0  TranslationZOffsetUnits=m
  Transform1 : sm_lib/Frames and Transforms/Rigid Transform  RotationMethod=ArbitraryAxis  FollAlignAxisA=+X  BaseAlignAxisA=+Y  FollAlignAxisB=+Y  BaseAlignAxisB=+Z  RotationStandardAxis=+Z  RotationAngle=1.9754511492118272  RotationAngleUnits=rad  RotationArbitraryAxis=[-0.53149434051907796 -0.53149434051907796 -0.65956616953295966]  RotationSequenceAxes=FollowerAxes  RotationSequence=XYX  RotationSequenceAngles=[0 0 0]  RotationSequenceAnglesUnits=deg  RotationMatrix=[1 0 0; 0 1 0; 0 0 1]  Quaternion=[1 0 0 0]  TranslationMethod=Cartesian  TranslationCartesianOffset=[-181.62772197331228 116.19029839316632 -133.82632242532665]  TranslationCartesianOffsetUnits=mm  TranslationStandardAxis=+Z  TranslationStandardOffset=0  TranslationStandardOffsetUnits=mm  TranslationROffset=0  TranslationROffsetUnits=m  TranslationThetaOffset=0  TranslationThetaOffsetUnits=deg  TranslationZOffset=0  TranslationZOffsetUnits=m
  Transform2 : sm_lib/Frames and Transforms/Rigid Transform  RotationMethod=ArbitraryAxis  FollAlignAxisA=+X  BaseAlignAxisA=+Y  FollAlignAxisB=+Y  BaseAlignAxisB=+Z  RotationStandardAxis=+Z  RotationAngle=2.0943951023931904  RotationAngleUnits=rad  RotationArbitraryAxis=[0.57735026918962595 0.57735026918962407 0.57735026918962729]  RotationSequenceAxes=FollowerAxes  RotationSequence=XYX  RotationSequenceAngles=[0 0 0]  RotationSequenceAnglesUnits=deg  RotationMatrix=[1 0 0; 0 1 0; 0 0 1]  Quaternion=[1 0 0 0]  TranslationMethod=Cartesian  TranslationCartesianOffset=[-186.51855936809574 126.39913469761754 -143.11837070915104]  TranslationCartesianOffsetUnits=mm  TranslationStandardAxis=+Z  TranslationStandardOffset=0  TranslationStandardOffsetUnits=mm  TranslationROffset=0  TranslationROffsetUnits=m  TranslationThetaOffset=0  TranslationThetaOffsetUnits=deg  TranslationZOffset=0  TranslationZOffsetUnits=m
  Transform3 : sm_lib/Frames and Transforms/Rigid Transform  RotationMethod=ArbitraryAxis  FollAlignAxisA=+X  BaseAlignAxisA=+Y  FollAlignAxisB=+Y  BaseAlignAxisB=+Z  RotationStandardAxis=+Z  RotationAngle=1.7850283121554718  RotationAngleUnits=rad  RotationArbitraryAxis=[1 8.1463180608813852e-16 -6.9713561493488163e-16]  RotationSequenceAxes=FollowerAxes  RotationSequence=XYX  RotationSequenceAngles=[0 0 0]  RotationSequenceAnglesUnits=deg  RotationMatrix=[1 0 0; 0 1 0; 0 0 1]  Quaternion=[1 0 0 0]  TranslationMethod=Cartesian  TranslationCartesianOffset=[-167.62772197331245 128.09991096385986 -150.93549038919824]  TranslationCartesianOffsetUnits=mm  TranslationStandardAxis=+Z  TranslationStandardOffset=0  TranslationStandardOffsetUnits=mm  TranslationROffset=0  TranslationROffsetUnits=m  TranslationThetaOffset=0  TranslationThetaOffsetUnits=deg  TranslationZOffset=0  TranslationZOffsetUnits=m
  Transform4 : sm_lib/Frames and Transforms/Rigid Transform  RotationMethod=ArbitraryAxis  FollAlignAxisA=+X  BaseAlignAxisA=+Y  FollAlignAxisB=+Y  BaseAlignAxisB=+Z  RotationStandardAxis=+Z  RotationAngle=1.5707963267948968  RotationAngleUnits=rad  RotationArbitraryAxis=[-5.5511151231257821e-17 -1 -5.5511151231257821e-17]  RotationSequenceAxes=FollowerAxes  RotationSequence=XYX  RotationSequenceAngles=[0 0 0]  RotationSequenceAnglesUnits=deg  RotationMatrix=[1 0 0; 0 1 0; 0 0 1]  Quaternion=[1 0 0 0]  TranslationMethod=Cartesian  TranslationCartesianOffset=[-167.62772197331239 126.39913469761737 -143.11837070915067]  TranslationCartesianOffsetUnits=mm  TranslationStandardAxis=+Z  TranslationStandardOffset=0  TranslationStandardOffsetUnits=mm  TranslationROffset=0  TranslationROffsetUnits=m  TranslationThetaOffset=0  TranslationThetaOffsetUnits=deg  TranslationZOffset=0  TranslationZOffsetUnits=m
  joint_1_RIGID : Subsystem
  F2 : PMIOPort  Side=Right
  F1 : PMIOPort  Port=2  Side=Left
  F : PMIOPort  Port=3  Side=Left
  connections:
  Transform/LConn1 -- ReferenceFrame/RConn1 -- Transform3/LConn1 -- Transform4/LConn1 -- Transform2/LConn1 -- Transform1/LConn1
  Transform/RConn1 -- F/RConn1
  Transform1/RConn1 -- F1/RConn1
  Transform2/RConn1 -- F2/RConn1
  Transform3/RConn1 -- joint_1_RIGID/LConn1
  AXE_BRAS_1_RIGID/LConn1 -- Transform4/RConn1

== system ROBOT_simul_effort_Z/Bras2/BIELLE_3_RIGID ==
  AXE_BIELLE_1_RIGID : Subsystem
  AXE_BIELLE_2_RIGID : Subsystem
  BIELLE_PARALLELOGRAMME_1_RIGID : Subsystem
  ReferenceFrame : sm_lib/Frames and Transforms/Reference Frame
  Transform : sm_lib/Frames and Transforms/Rigid Transform  RotationMethod=ArbitraryAxis  FollAlignAxisA=+X  BaseAlignAxisA=+Y  FollAlignAxisB=+Y  BaseAlignAxisB=+Z  RotationStandardAxis=+Z  RotationAngle=2.0943951023931957  RotationAngleUnits=rad  RotationArbitraryAxis=[-0.57735026918962584 -0.57735026918962573 -0.57735026918962573]  RotationSequenceAxes=FollowerAxes  RotationSequence=XYX  RotationSequenceAngles=[0 0 0]  RotationSequenceAnglesUnits=deg  RotationMatrix=[1 0 0; 0 1 0; 0 0 1]  Quaternion=[1 0 0 0]  TranslationMethod=Cartesian  TranslationCartesianOffset=[-181.12877100137212 -3.0000000000000853 -105.74999999999531]  TranslationCartesianOffsetUnits=mm  TranslationStandardAxis=+Z  TranslationStandardOffset=0  TranslationStandardOffsetUnits=mm  TranslationROffset=0  TranslationROffsetUnits=m  TranslationThetaOffset=0  TranslationThetaOffsetUnits=deg  TranslationZOffset=0  TranslationZOffsetUnits=m
  Transform1 : sm_lib/Frames and Transforms/Rigid Transform  RotationMethod=ArbitraryAxis  FollAlignAxisA=+X  BaseAlignAxisA=+Y  FollAlignAxisB=+Y  BaseAlignAxisB=+Z  RotationStandardAxis=+Z  RotationAngle=2.0943951023931953  RotationAngleUnits=rad  RotationArbitraryAxis=[0.57735026918962584 -0.57735026918962584 0.57735026918962584]  RotationSequenceAxes=FollowerAxes  RotationSequence=XYX  RotationSequenceAngles=[0 0 0]  RotationSequenceAnglesUnits=deg  RotationMatrix=[1 0 0; 0 1 0; 0 0 1]  Quaternion=[1 0 0 0]  TranslationMethod=Cartesian  TranslationCartesianOffset=[-181.12877100136708 12.999999999999984 -3.2500000000000027]  TranslationCartesianOffsetUnits=mm  TranslationStandardAxis=+Z  TranslationStandardOffset=0  TranslationStandardOffsetUnits=mm  TranslationROffset=0  TranslationROffsetUnits=m  TranslationThetaOffset=0  TranslationThetaOffsetUnits=deg  TranslationZOffset=0  TranslationZOffsetUnits=m
  Transform2 : sm_lib/Frames and Transforms/Rigid Transform  RotationMethod=ArbitraryAxis  FollAlignAxisA=+X  BaseAlignAxisA=+Y  FollAlignAxisB=+Y  BaseAlignAxisB=+Z  RotationStandardAxis=+Z  RotationAngle=3.1415926535897931  RotationAngleUnits=rad  RotationArbitraryAxis=[-0.70710678118654746 0.70710678118654757 0]  RotationSequenceAxes=FollowerAxes  RotationSequence=XYX  RotationSequenceAngles=[0 0 0]  RotationSequenceAnglesUnits=deg  RotationMatrix=[1 0 0; 0 1 0; 0 0 1]  Quaternion=[1 0 0 0]  TranslationMethod=Cartesian  TranslationCartesianOffset=[-178.12877100136706 4.9999999999999902 -54.499999999999957]  TranslationCartesianOffsetUnits=mm  TranslationStandardAxis=+Z  TranslationStandardOffset=0  TranslationStandardOffsetUnits=mm  TranslationROffset=0  TranslationROffsetUnits=m  TranslationThetaOffset=0  TranslationThetaOffsetUnits=deg  TranslationZOffset=0  TranslationZOffsetUnits=m
  Transform3 : sm_lib/Frames and Transforms/Rigid Transform  RotationMethod=ArbitraryAxis  FollAlignAxisA=+X  BaseAlignAxisA=+Y  FollAlignAxisB=+Y  BaseAlignAxisB=+Z  RotationStandardAxis=+Z  RotationAngle=1.7602050674842991  RotationAngleUnits=rad  RotationArbitraryAxis=[-0.82650316451596495 -0.3980530863120495 -0.3980530863120495]  RotationSequenceAxes=FollowerAxes  RotationSequence=XYX  RotationSequenceAngles=[0 0 0]  RotationSequenceAnglesUnits=deg  RotationMatrix=[1 0 0; 0 1 0; 0 0 1]  Quaternion=[1 0 0 0]  TranslationMethod=Cartesian  TranslationCartesianOffset=[-181.12877100136708 4.9999999999999627 -105.74999999999996]  TranslationCartesianOffsetUnits=mm  TranslationStandardAxis=+Z  TranslationStandardOffset=0  TranslationStandardOffsetUnits=mm  TranslationROffset=0  TranslationROffsetUnits=m  TranslationThetaOffset=0  TranslationThetaOffsetUnits=deg  TranslationZOffset=0  TranslationZOffsetUnits=m
  Transform4 : sm_lib/Frames and Transforms/Rigid Transform  RotationMethod=ArbitraryAxis  FollAlignAxisA=+X  BaseAlignAxisA=+Y  FollAlignAxisB=+Y  BaseAlignAxisB=+Z  RotationStandardAxis=+Z  RotationAngle=1.7602050674842997  RotationAngleUnits=rad  RotationArbitraryAxis=[-0.82650316451596506 -0.39805308631204933 -0.39805308631204928]  RotationSequenceAxes=FollowerAxes  RotationSequence=XYX  RotationSequenceAngles=[0 0 0]  RotationSequenceAnglesUnits=deg  RotationMatrix=[1 0 0; 0 1 0; 0 0 1]  Quaternion=[1 0 0 0]  TranslationMethod=Cartesian  TranslationCartesianOffset=[-181.12877100136708 4.9999999999999627 -3.2500000000000027]  TranslationCartesianOffsetUnits=mm  TranslationStandardAxis=+Z  TranslationStandardOffset=0  TranslationStandardOffsetUnits=mm  TranslationROffset=0  TranslationROffsetUnits=m  TranslationThetaOffset=0  TranslationThetaOffsetUnits=deg  TranslationZOffset=0  TranslationZOffsetUnits=m
  F : PMIOPort  Side=Left
  F1 : PMIOPort  Port=2  Side=Right
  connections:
  Transform/LConn1 -- ReferenceFrame/RConn1 -- Transform3/LConn1 -- Transform4/LConn1 -- Transform2/LConn1 -- Transform1/LConn1
  Transform/RConn1 -- F/RConn1
  Transform1/RConn1 -- F1/RConn1
  BIELLE_PARALLELOGRAMME_1_RIGID/LConn1 -- Transform2/RConn1
  AXE_BIELLE_1_RIGID/LConn1 -- Transform3/RConn1
  AXE_BIELLE_2_RIGID/LConn1 -- Transform4/RConn1

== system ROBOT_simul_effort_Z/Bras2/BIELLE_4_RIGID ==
  AXE_BIELLE_1_RIGID : Subsystem
  AXE_BIELLE_2_RIGID : Subsystem
  BIELLE_PARALLELOGRAMME_1_RIGID : Subsystem
  ReferenceFrame : sm_lib/Frames and Transforms/Reference Frame
  Transform : sm_lib/Frames and Transforms/Rigid Transform  RotationMethod=ArbitraryAxis  FollAlignAxisA=+X  BaseAlignAxisA=+Y  FollAlignAxisB=+Y  BaseAlignAxisB=+Z  RotationStandardAxis=+Z  RotationAngle=2.0943951023931948  RotationAngleUnits=rad  RotationArbitraryAxis=[0.57735026918962562 -0.57735026918962706 0.57735026918962473]  RotationSequenceAxes=FollowerAxes  RotationSequence=XYX  RotationSequenceAngles=[0 0 0]  RotationSequenceAnglesUnits=deg  RotationMatrix=[1 0 0; 0 1 0; 0 0 1]  Quaternion=[1 0 0 0]  TranslationMethod=Cartesian  TranslationCartesianOffset=[-181.12877100136237 13.000000000000043 -105.74999999999874]  TranslationCartesianOffsetUnits=mm  TranslationStandardAxis=+Z  TranslationStandardOffset=0  TranslationStandardOffsetUnits=mm  TranslationROffset=0  TranslationROffsetUnits=m  TranslationThetaOffset=0  TranslationThetaOffsetUnits=deg  TranslationZOffset=0  TranslationZOffsetUnits=m
  Transform1 : sm_lib/Frames and Transforms/Rigid Transform  RotationMethod=ArbitraryAxis  FollAlignAxisA=+X  BaseAlignAxisA=+Y  FollAlignAxisB=+Y  BaseAlignAxisB=+Z  RotationStandardAxis=+Z  RotationAngle=2.0943951023931953  RotationAngleUnits=rad  RotationArbitraryAxis=[0.57735026918962584 -0.57735026918962562 0.57735026918962595]  RotationSequenceAxes=FollowerAxes  RotationSequence=XYX  RotationSequenceAngles=[0 0 0]  RotationSequenceAnglesUnits=deg  RotationMatrix=[1 0 0; 0 1 0; 0 0 1]  Quaternion=[1 0 0 0]  TranslationMethod=Cartesian  TranslationCartesianOffset=[-181.12877100136717 13 -3.2500000000000062]  TranslationCartesianOffsetUnits=mm  TranslationStandardAxis=+Z  TranslationStandardOffset=0  TranslationStandardOffsetUnits=mm  TranslationROffset=0  TranslationROffsetUnits=m  TranslationThetaOffset=0  TranslationThetaOffsetUnits=deg  TranslationZOffset=0  TranslationZOffsetUnits=m
  Transform2 : sm_lib/Frames and Transforms/Rigid Transform  RotationMethod=ArbitraryAxis  FollAlignAxisA=+X  BaseAlignAxisA=+Y  FollAlignAxisB=+Y  BaseAlignAxisB=+Z  RotationStandardAxis=+Z  RotationAngle=3.1415926535897931  RotationAngleUnits=rad  RotationArbitraryAxis=[-0.70710678118654746 0.70710678118654757 -3.9252311467094373e-17]  RotationSequenceAxes=FollowerAxes  RotationSequence=XYX  RotationSequenceAngles=[0 0 0]  RotationSequenceAnglesUnits=deg  RotationMatrix=[1 0 0; 0 1 0; 0 0 1]  Quaternion=[1 0 0 0]  TranslationMethod=Cartesian  TranslationCartesianOffset=[-178.12877100136717 5.0000000000000044 -54.5]  TranslationCartesianOffsetUnits=mm  TranslationStandardAxis=+Z  TranslationStandardOffset=0  TranslationStandardOffsetUnits=mm  TranslationROffset=0  TranslationROffsetUnits=m  TranslationThetaOffset=0  TranslationThetaOffsetUnits=deg  TranslationZOffset=0  TranslationZOffsetUnits=m
  Transform3 : sm_lib/Frames and Transforms/Rigid Transform  RotationMethod=ArbitraryAxis  FollAlignAxisA=+X  BaseAlignAxisA=+Y  FollAlignAxisB=+Y  BaseAlignAxisB=+Z  RotationStandardAxis=+Z  RotationAngle=1.7602050674842993  RotationAngleUnits=rad  RotationArbitraryAxis=[-0.82650316451596484 -0.39805308631204944 -0.39805308631204939]  RotationSequenceAxes=FollowerAxes  RotationSequence=XYX  RotationSequenceAngles=[0 0 0]  RotationSequenceAnglesUnits=deg  RotationMatrix=[1 0 0; 0 1 0; 0 0 1]  Quaternion=[1 0 0 0]  TranslationMethod=Cartesian  TranslationCartesianOffset=[-181.1287710013672 5.0000000000000044 -105.75000000000003]  TranslationCartesianOffsetUnits=mm  TranslationStandardAxis=+Z  TranslationStandardOffset=0  TranslationStandardOffsetUnits=mm  TranslationROffset=0  TranslationROffsetUnits=m  TranslationThetaOffset=0  TranslationThetaOffsetUnits=deg  TranslationZOffset=0  TranslationZOffsetUnits=m
  Transform4 : sm_lib/Frames and Transforms/Rigid Transform  RotationMethod=ArbitraryAxis  FollAlignAxisA=+X  BaseAlignAxisA=+Y  FollAlignAxisB=+Y  BaseAlignAxisB=+Z  RotationStandardAxis=+Z  RotationAngle=1.7602050674842997  RotationAngleUnits=rad  RotationArbitraryAxis=[-0.82650316451596506 -0.39805308631204939 -0.39805308631204916]  RotationSequenceAxes=FollowerAxes  RotationSequence=XYX  RotationSequenceAngles=[0 0 0]  RotationSequenceAnglesUnits=deg  RotationMatrix=[1 0 0; 0 1 0; 0 0 1]  Quaternion=[1 0 0 0]  TranslationMethod=Cartesian  TranslationCartesianOffset=[-181.12877100136717 5.0000000000000044 -3.2500000000000027]  TranslationCartesianOffsetUnits=mm  TranslationStandardAxis=+Z  TranslationStandardOffset=0  TranslationStandardOffsetUnits=mm  TranslationROffset=0  TranslationROffsetUnits=m  TranslationThetaOffset=0  TranslationThetaOffsetUnits=deg  TranslationZOffset=0  TranslationZOffsetUnits=m
  F : PMIOPort  Side=Left
  F1 : PMIOPort  Port=2  Side=Right
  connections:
  Transform/LConn1 -- ReferenceFrame/RConn1 -- Transform3/LConn1 -- Transform4/LConn1 -- Transform2/LConn1 -- Transform1/LConn1
  Transform/RConn1 -- F/RConn1
  Transform1/RConn1 -- F1/RConn1
  BIELLE_PARALLELOGRAMME_1_RIGID/LConn1 -- Transform2/RConn1
  AXE_BIELLE_1_RIGID/LConn1 -- Transform3/RConn1
  AXE_BIELLE_2_RIGID/LConn1 -- Transform4/RConn1

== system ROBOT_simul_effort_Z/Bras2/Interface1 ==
  Angular Velocity Source : fl_lib/Mechanical/Mechanical Sources/Ideal Angular Velocity Source
  Torque Sensor : fl_lib/Mechanical/Mechanical Sensors/Ideal Torque Sensor
  C : PMIOPort  Side=Left
  T : PMIOPort  Port=2  Side=Right
  w : PMIOPort  Port=3  Side=Right
  R : PMIOPort  Port=4  Side=Left
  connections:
  Angular Velocity Source/RConn1 -- w/RConn1
  C/RConn1 -- Torque Sensor/RConn1
  Torque Sensor/RConn2 -- T/RConn1
  Torque Sensor/LConn1 -- Angular Velocity Source/RConn2
  R/RConn1 -- Angular Velocity Source/LConn1
